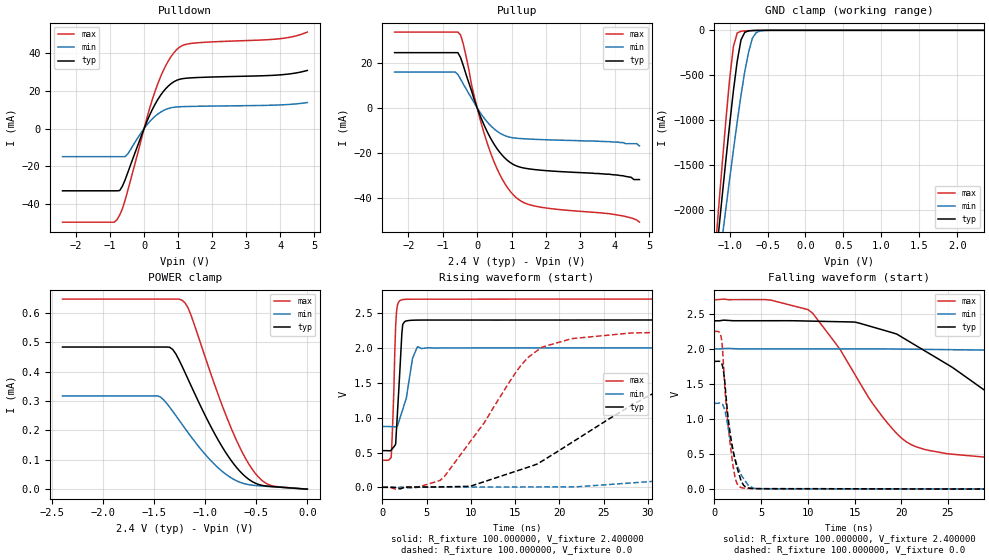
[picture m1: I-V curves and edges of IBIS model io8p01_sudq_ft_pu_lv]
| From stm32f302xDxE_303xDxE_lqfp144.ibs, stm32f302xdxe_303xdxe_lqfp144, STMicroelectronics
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|   Model io8p01_sudq_ft_pu_lv
[Model]  io8p01_sudq_ft_pu_lv
Model_type I/O
Polarity   Non-Inverting
Enable   Active-Low
Vinl =   0.720000V
Vinh =   1.680000V
Vmeas =  1.200000V
Cref =   50.000000pF
Rref =   100.000000M
Vref =   0.0V
C_comp   1.970100pF   1.887900pF   2.069400pF
[Temperature Range]   25.000000   0.125000k   -40.000000
[Pullup Reference]   2.400000V   2.000000V   2.700000V
[Pulldown Reference]   0.0V   0.0V   0.0V
[POWER Clamp Reference]   2.400000V   2.000000V   2.700000V
[GND Clamp Reference]   0.0V   0.0V   0.0V
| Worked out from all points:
|   slope of the pulldown table from 0 to 0.36 V, typ, clamps not added: 25.5 ohm
|   slope of the pullup table from 0 to 0.36 V, typ, clamps not added: 28.4 ohm
|   GND clamp passes 1 mA (typ) near -0.64 V on its own axis
|   rising waveform, R_fixture 100.000000, V_fixture 2.400000: 20-80 % time 497ps typ, 1.06ns min, 335ps max; typ from 0.527 V to 2.4 V
|   rising waveform, R_fixture 100.000000, V_fixture 0.0: 20-80 % time 14.6ns typ, 42.8ns min, 7.27ns max; typ from 0.001 V to 1.82 V
|   falling waveform, R_fixture 100.000000, V_fixture 2.400000: 20-80 % time 12.9ns typ, 32.5ns min, 7.06ns max; typ from 2.4 V to 0.527 V
|   falling waveform, R_fixture 100.000000, V_fixture 0.0: 20-80 % time 1.16ns typ, 1.4ns min, 913ps max; typ from 1.82 V to 0.001 V
[Pulldown]
|Voltage   I(typ)   I(min)   I(max)
-2.4V     -33.16mA   -14.98mA   -49.86mA
-880mV    -33.16mA   -14.98mA   -49.86mA
-800mV    -33.16mA   -14.98mA   -48.55mA
-640mV    -30.75mA   -14.98mA   -42.77mA
-480mV    -23.43mA   -13.57mA   -32.92mA
80mV      3.651mA    1.905mA    5.506mA
400mV     15.37mA    7.665mA    23.73mA
720mV     22.75mA    10.69mA    36.23mA
1.04V     26.18mA    11.57mA    43.27mA
1.52V     27.09mA    11.81mA    45.55mA
4V        28.55mA    12.55mA    47.81mA
4.8V      30.9mA     13.81mA    51.31mA
[Pullup]
|Voltage   I(typ)   I(min)   I(max)
-2.4V     24.57mA    15.91mA    33.73mA
-640mV    24.57mA    15.91mA    33.73mA
-480mV    22.32mA    12.71mA    32.43mA
-400mV    18.71mA    10.52mA    28.28mA
-160mV    7.421mA    4.162mA    10.02mA
0V        81fA       15.2pA     0A
320mV     -11.51mA   -6.781mA   -16.98mA
720mV     -21mA      -11.8mA    -31.53mA
1.2V      -26.24mA   -13.65mA   -40.83mA
1.76V     -27.69mA   -14.12mA   -44.07mA
3.84V     -29.6mA    -15.1mA    -47.2mA
4.72V     -32mA      -17mA      -51mA
[GND_clamp]
|Voltage   I(typ)   I(min)   I(max)
-2.4V     -9.788A    -9.782A    -9.734A
-1.2V     -2.718A    -3.02A     -2.568A
-1.15V    -2.29A     -2.675A    -2.036A
-1.1V     -1.868A    -2.333A    -1.515A
-1.05V    -1.454A    -1.995A    -1.012A
-950mV    -674.5mA   -1.337A    -180.5mA
-900mV    -345.2mA   -1.023A    -29.72mA
-850mV    -106.4mA   -726mA     -10.13mA
-750mV    -6.396mA   -244mA     -4.026mA
-700mV    -2.558mA   -88.61mA   -2.329mA
-600mV    -416uA     -7.739mA   -368uA
2.35V     0A         0A         0A
[POWER_clamp]
|Voltage   I(typ)   I(min)   I(max)
-2.4V     483.8uA    317.4uA    647uA
-1.47V    483.8uA    317.4uA    647uA
-1.32V    475.6uA    265.2uA    647uA
-1.23V    419.7uA    221.6uA    643.3uA
-1.17V    374.8uA    192.7uA    617.6uA
-1.14V    352.1uA    178.7uA    591.9uA
-840mV    147uA      62.15uA    289.6uA
-690mV    72.24uA    27.76uA    162.7uA
-540mV    25.74uA    13.55uA    67.63uA
-450mV    13.38uA    10.75uA    31.36uA
-360mV    9.231uA    8.535uA    12.97uA
0V        0A         0A         0A
[Ramp]
| variable   typ   min   max
dV/dt_r  1.09269/14.55881n   0.73353/42.71845n   1.34908/7.26325n
dV/dt_f  1.12400/12.83842n   0.67649/32.44923n   1.38689/7.04961n
R_load = 100.000000
[Rising Waveform]
R_fixture= 100.000000
V_fixture= 2.400000
V_fixture_min= 2.000000
V_fixture_max= 2.700000
|time   V(typ)   V(min)   V(max)
0s        526.5mV    872.5mV    388.6mV
1.001ns   534.8mV    870.7mV    429.3mV
1.301ns   581.8mV    869.1mV    1.401V
1.502ns   620.7mV    868.5mV    2.316V
1.602ns   841mV      868.2mV    2.522V
2.102ns   1.968V     1.038V     2.685V
2.302ns   2.337V     1.118V     2.692V
3.403ns   2.396V     1.846V     2.698V
4.004ns   2.398V     2.018V     2.698V
49.85ns   2.4V       2V         2.7V
[Rising Waveform]
R_fixture= 100.000000
V_fixture= 0.0
V_fixture_min= 0.0
V_fixture_max= 0.0
|time   V(typ)   V(min)   V(max)
0s        1.057mV    1.357mV    941.6uV
6.507ns   6.739mV    4.851mV    98.8mV
15.52ns   249.4mV    5.766mV    1.725V
18.02ns   374.6mV    6.657mV    2.009V
28.03ns   1.166V     62.6mV     2.213V
34.53ns   1.553V     120.9mV    2.23V
43.04ns   1.725V     229mV      2.248V
79.08ns   1.822V     883.8mV    2.25V
103.1ns   1.822V     1.116V     2.249V
249.2ns   1.822V     1.224V     2.25V
[Falling Waveform]
R_fixture= 100.000000
V_fixture= 2.400000
V_fixture_min= 2.000000
V_fixture_max= 2.700000
|time   V(typ)   V(min)   V(max)
0s        2.4V       2V         2.7V
10.01ns   2.397V     2V         2.56V
15.02ns   2.383V     2V         1.64V
20.02ns   2.171V     1.997V     729.2mV
29.53ns   1.353V     1.982V     451.1mV
38.04ns   762.8mV    1.926V     413.2mV
57.06ns   576.4mV    1.555V     391.8mV
84.58ns   537.8mV    1.049V     388.5mV
102.6ns   530.3mV    958.5mV    388.5mV
249.2ns   526.5mV    872.5mV    388.6mV
[Falling Waveform]
R_fixture= 100.000000
V_fixture= 0.0
V_fixture_min= 0.0
V_fixture_max= 0.0
|time   V(typ)   V(min)   V(max)
0s        1.822V     1.224V     2.25V
700.7ps   1.803V     1.224V     2.18V
800.8ps   1.785V     1.217V     2.098V
1.001ns   1.655V     1.167V     1.705V
1.401ns   1.091V     924.7mV    994.1mV
1.802ns   692.7mV    650.1mV    517.8mV
2.302ns   370.4mV    389.6mV    121.1mV
2.903ns   110.3mV    193.7mV    21.86mV
4.605ns   7.762mV    8.133mV    8.175mV
49.85ns   1.057mV    1.357mV    941.6uV
